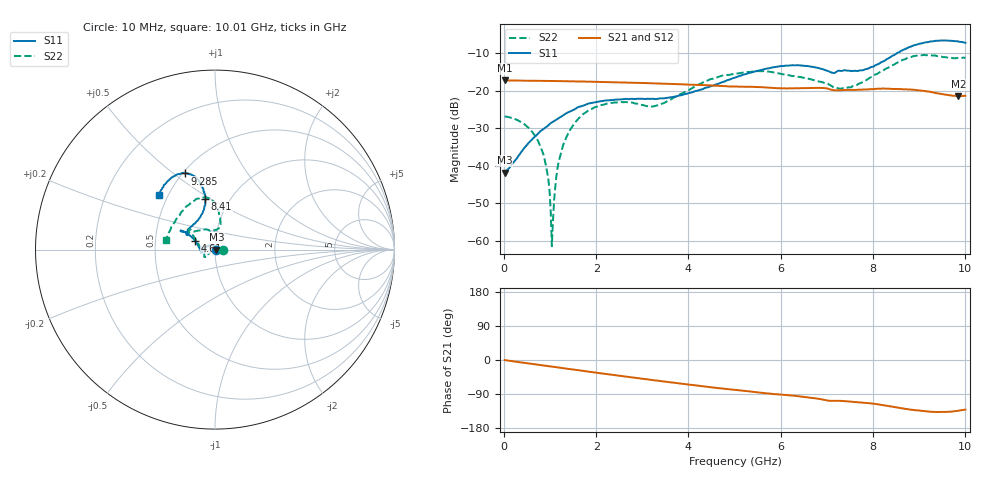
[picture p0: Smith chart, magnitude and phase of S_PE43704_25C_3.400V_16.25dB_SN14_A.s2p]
! Device ID: PE43704
! Dir: z:\PE43704\PE43704_Char_1_20130516\PE43704\AMB\3p400V\16p25dB
! Serial: 14
! Insertion: A
! Impedance: 50 ohm
! Temp: Amb
! VDD: 3.400V
! Attenuation Step: 16.25dB
! IDD: 1.139829e-01mA
#  Hz  S  RI  R  50
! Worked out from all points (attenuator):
!   401 points, 10 MHz to 10.01 GHz, reference 50 ohm
!   highest |S21| = -17.23 dB at 10 MHz (marker M1); lowest = -21.4 dB at 9.86 GHz (marker M2)
!   lowest |S11| = -41.8 dB at 10 MHz (marker M3), VSWR 1.02, Z = 50.8 + j0.0411 ohm
!   |S11| at or under -10 dB: start of sweep to 8.522 GHz
!   |S22| runs from -61.4 to -10.4 dB; largest |S21 - S12| = 0.0015
!   S11 on the Smith chart (normalised r, x): 10 MHz: 1.02, +0.00; 4.61 GHz: 0.79, +0.08; 8.41 GHz: 0.77, +0.48; 9.285 GHz: 0.51, +0.55; 10.01 GHz: 0.45, +0.34
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1e7  0.00814 0.000404  0.1376 -0.000431  0.1376 -0.000398  0.0454 -2.49e-05
4.35e8  0.00115 0.0172  0.1352 -0.0178  0.1354 -0.0179  0.0355 0.0062
7.35e8  -0.0118 0.0242  0.1327 -0.0296  0.1327 -0.0295  0.0207 0.00569
9.1e8  -0.0217 0.0246  0.1306 -0.0362  0.1307 -0.0361  0.00956 0.00269
1.01e9  -0.0277 0.0247  0.1294 -0.0399  0.1293 -0.0399  0.0025 0.000399
1.035e9  -0.0293 0.0242  0.1291 -0.0409  0.129 -0.0407  0.000589 -0.000614
1.085e9  -0.0319 0.0234  0.1283 -0.0427  0.1283 -0.0427  -0.00261 -0.00234
1.16e9  -0.0362 0.0222  0.1271 -0.0455  0.1271 -0.0454  -0.00814 -0.00497
1.26e9  -0.0417 0.0202  0.1253 -0.0491  0.1254 -0.0491  -0.015 -0.00834
1.435e9  -0.051 0.0149  0.1222 -0.055  0.1221 -0.055  -0.0259 -0.0161
1.685e9  -0.0622 0.00648  0.1171 -0.0633  0.1171 -0.0633  -0.0388 -0.027
2.36e9  -0.0743 -0.0141  0.1008 -0.0825  0.1008 -0.0824  -0.0554 -0.042
3.36e9  -0.0784 -0.0108  0.0716 -0.1026  0.0717 -0.1026  -0.0641 -0.00635
4.61e9  -0.1121 0.0497  0.0328 -0.1122  0.033 -0.1121  -0.1268 0.0819
5.01e9  -0.132 0.0714  0.0223 -0.1119  0.0225 -0.1121  -0.1412 0.0926
6.685e9  -0.1843 0.1002  -0.0189 -0.1077  -0.019 -0.1076  -0.0933 0.1057
7.385e9  -0.1515 0.1115  -0.0326 -0.0975  -0.0326 -0.0973  -0.00598 0.1072
8.36e9  -0.054 0.27  -0.0562 -0.0906  -0.0561 -0.0908  0.0221 0.2066
8.41e9  -0.0545 0.2839  -0.0577 -0.0892  -0.0575 -0.0896  0.017 0.2161
9.285e9  -0.1663 0.4242  -0.0698 -0.0657  -0.0699 -0.0653  -0.1137 0.2733
9.86e9  -0.2875 0.35  -0.0587 -0.0612  -0.059 -0.0606  -0.2457 0.1176
1.001e10  -0.3118 0.306  -0.0564 -0.0649  -0.0572 -0.0651  -0.2712 0.0559
